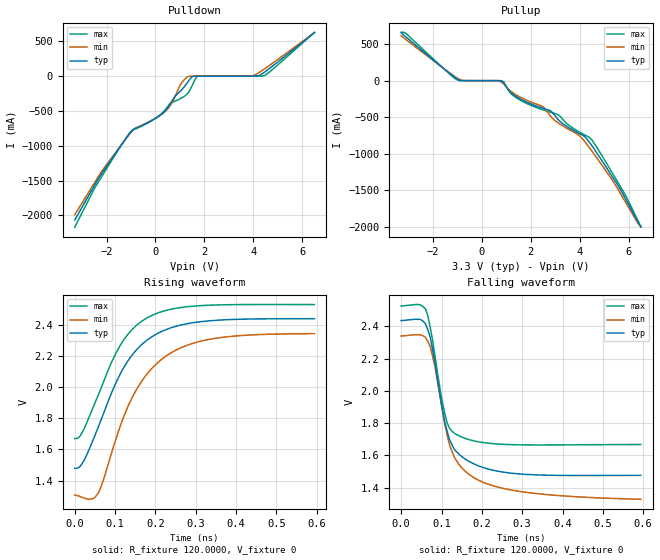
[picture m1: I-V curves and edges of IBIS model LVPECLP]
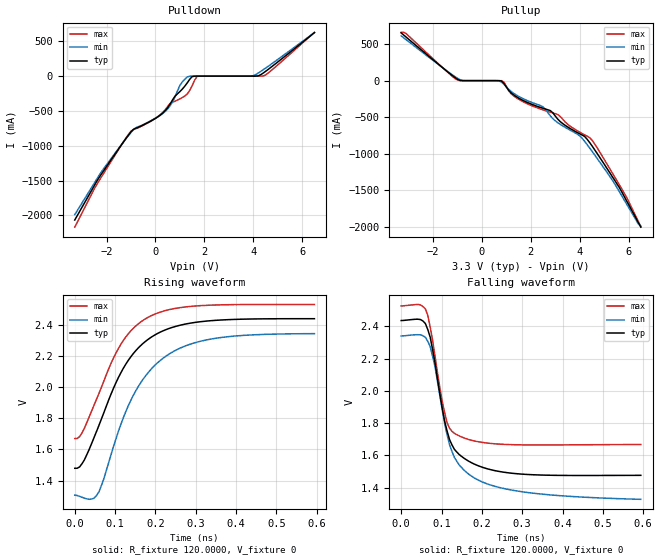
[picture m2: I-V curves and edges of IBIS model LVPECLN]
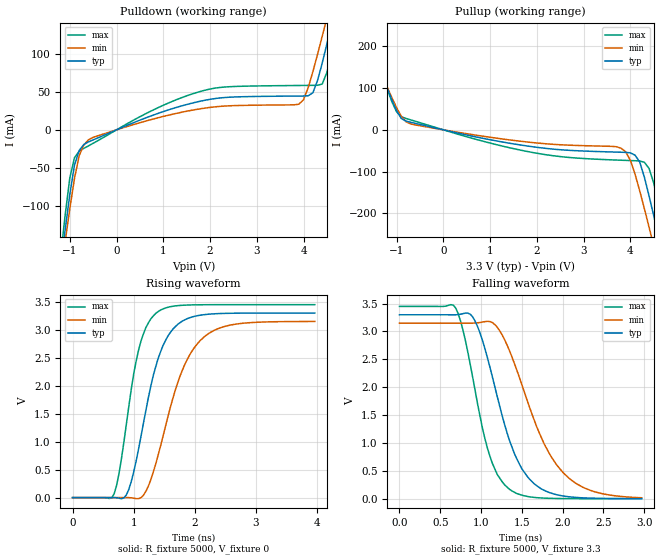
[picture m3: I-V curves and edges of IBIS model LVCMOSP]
|   National Semiconductor Corporation
|   IBIS Model of LMK04000
[IBIS Ver]   4.0
[File name]   lmk04000.ibs
[File Rev]   1.1
[Notes]
 Created By  Shrikant G Kadadevar, Pegah Alavi
   Revision History
   1.0   | Initial Release (SK)
   1.1   | Updated package model per designer's request (PA)
   | Updated pin names & numbers per designer's request (PA)
   | Changed IBIS version from 3.2 to 4.0  (PA)
[Date]   07/09/2009
[Source]  Generated by National Semincoductor Corporation.
[Disclaimer]
(C) Copyright National Semiconductor Corporation 2009
   All rights reserved
National Semiconductor Corporation hereby grants the
user of this IBIS model a non-exclusive, nontransferable
license to use this IBIS model under the following terms.
Before using this IBIS model, the user should read this
license.  If the user does not accept these terms,  the
IBIS model should be returned to National within 30 days.
The user is granted this license only to use the
IBIS model and is not granted rights to sell, load, rent,
lease or license the IBIS model in whole or in part, or in
modified form to anyone other than user. User may modify
the IBIS model to suit its specific applications but rights
to derivative works and such modifications shall belong to
National.
This IBIS model is provided on an "AS IS" basis and
National makes absolutely no warranty with respect to the
information contained herein.NATIONAL DISCLAIMS AND CUSTOMER
WAIVES ALL WARRANTIES, EXPRESS OR IMPLIED, INCLUDING
WARRANTIES OF MERCHANTABILITY OR FITNESS FOR A PARTICULAR
PURPOSE. The entire risk as to quality and performance is
with the Customer. ACCORDINGLY, IN NO EVENT SHALL THE
COMPANY BE LIABLE FOR ANY DAMAGES, WHETHER IN CONTRACT OR
TORT,INCLUDING ANY LOST PROFITS OR OTHER INCIDENTAL,
CONSEQUENTIAL, EXEMPLARY, OR PUNITIVE DAMAGES ARISING OUT
OF THE USE OR APPLICATION OF THE IBIS model provided in
this package.Further, National reserves the right to make
changes without notice to any product herein to improve
reliability, function, or design. National does not convey
any license under patent rights or any other intellectual
property rights, including those of third parties.
National is not obligated to provide maintenance or support
for the licensed IBIS model.
[Copyright]  Copyright 2009, National Semiconductor, All Rights Reserved
[Component]  LMK04000
[Manufacturer]  National Semiconductor Corp
[Package]
|   typ   min   max
R_pkg   0   0   0
L_pkg   0   0   0
C_pkg   0   0   0
[Pin]   signal_name   model_name   R_pin   L_pin   C_pin
1   GND   GND
2   FOUT   NC
3   VCC1   POWER
4   CLKUWIRE   NC
5   DATAUWIRE   NC
6   LEUWIRE   NC
7   NC   NC
8   VCC2   POWER
9   LDOBYP1   POWER
10   LDOBYP2   POWER
11   GOE   NC
12   LD   NC
13   VCC3   POWER
14   CLKOUT0   LVPECLP
15   CLKOUT0*   LVPECLN
16   DLD_BYP   NC
17   GND   POWER
18   VCC4   POWER
19   VCC5   POWER
20   CLKIN0   CLKINP
21   CLKIN0*   CLKINN
22   VCC6   POWER
23   CPOUT1   NC
24   VCC7   POWER
25   CLKIN1   CLKINP
26   CLKIN1*   CLKINN
27   SYNC*   NC
28   OSCIN   OSCINP
29   OSCIN*   OSCINN
30   VCC8   POWER
31   VCC9   POWER
32   CPOUT2   NC
33   VCC10   POWER
34   CLKIN0_LOS   NC
35   CLKIN1_LOS   NC
36   BIAS   NC
37   VCC11   POWER
38   CLKOUT1   LVPECLP
39   CLKOUT1*   LVPECLN
40   VCC12   POWER
41   CLKOUT2   LVCMOSP
42   CLKOUT2*   LVCMOSN
43   VCC13   POWER
44   CLKOUT3   LVCMOSP
45   CLKOUT3*   LVCMOSN
46   VCC14   POWER
47   CLKOUT4   LVPECLP
48   CLKOUT4*   LVPECLN
49   DAP   GND
[Diff pin]  inv_pin  vdiff  tdelay_typ  tdelay_min  tdelay_max
14   15   0.0   0.0s   0.0s   0.0s
20   21   300m   0.0s   0.0s   0.0s
25   26   300m   0.0s   0.0s   0.0s
28   29   300m   0.0s   0.0s   0.0s
38   39   0.0   0.0s   0.0s   0.0s
41   42   0.0   0.0s   0.0s   0.0s
44   45   0.0   0.0s   0.0s   0.0s
47   48   0.0   0.0s   0.0s   0.0s
[Package Model] llp48_lmk04000bisq
[Define Package Model]  llp48_lmk04000bisq
[Manufacturer]  Unknown
[OEM]  Unknown
[Description]  48 LLP for LMK04000 (5GHz simulation Frequency)
[Number Of Pins]  49
[Pin Numbers]
1   | 1 = L1
2   | 2 = L2
3   | 3 = L3
4   | 4 = L4
5   | 5 = L5
6   | 6 = L6
7   | 7 = L7
8   | 8 = L8
9   | 9 = L9
10   | 10 = L10
11   | 11 = L11
12   | 12 = L12
13   | 13 = L13
14   | 14 = L14
15   | 15 = L15
16   | 16 = L16
17   | 17 = L17
18   | 18 = L18
19   | 19 = L19
20   | 20 = L20
21   | 21 = L21
22   | 22 = L22
23   | 23 = L23
24   | 24 = L24
25   | 25 = L25
26   | 26 = L26
27   | 27 = L27
28   | 28 = L28
29   | 29 = L29
30   | 30 = L30
31   | 31 = L31
32   | 32 = L32
33   | 33 = L33
34   | 34 = L34
35   | 35 = L35
36   | 36 = L36
37   | 37 = L37
38   | 38 = L38
39   | 39 = L39
40   | 40 = L40
41   | 41 = L41
42   | 42 = L42
43   | 43 = L43
44   | 44 = L44
45   | 45 = L45
46   | 46 = L46
47   | 47 = L47
48   | 48 = L48
49   | 49 = LDAP
[Model Data]
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[End Model Data]
[End Package Model]
| Models and submodels in the file (8): LVPECLP (Output), LVPECLN (Output), LVCMOSP (Output), LVCMOSN (Output), OSCINP (Input), OSCINN (Input), CLKINP (Input), CLKINN (Input)
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|   Model LVPECLP
[Model]  LVPECLP
Model_type Output
Polarity   Non-Inverting
Vmeas =  1.9572
Rref =   120.0000
Vref =   0
C_comp   1.5000pF   NA   NA
[Temperature Range]   25.0000   85.0000   -40.0000
[Voltage Range]   3.3000V   3.1500V   3.4500V
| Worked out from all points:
|   slope of the pulldown table from 0 to 0.495 V, typ, clamps not added: 3.28 ohm
|   rising waveform, R_fixture 120.0000, V_fixture 0: 20-80 % time 109ps typ, 113ps min, 97ps max; typ from 1.48 V to 2.44 V
|   falling waveform, R_fixture 120.0000, V_fixture 0: 20-80 % time 46.6ps typ, 63.2ps min, 35.4ps max; typ from 2.44 V to 1.48 V
[Pulldown]
|Voltage   I(typ)   I(min)   I(max)
-3.3V     -2.068A    -1.991A    -2.17A
-2.4V     -1.51A     -1.48A     -1.557A
-1V       -800.1mA   -808.9mA   -790.6mA
400mV     -496mA     -506.6mA   -482.6mA
700mV     -340.5mA   -370.2mA   -374.4mA
1V        -221.6mA   -133.2mA   -327mA
1.3V      -96.95mA   -12.44mA   -256.5mA
1.5V      -7.042mA   -45.2uA    -138.2mA
1.7V      -4.607uA   -80.81nA   -4.382mA
4V        8.686uA    6.676mA    32.57pA
4.5V      67.89mA    114.4mA    16.63mA
6.5V      624.9mA    626mA      629.5mA
[Pullup]
|Voltage   I(typ)   I(min)   I(max)
-3.3V     653.2mA    613mA      661mA
-3.1V     596.5mA    561.2mA    645.3mA
-1V       19.76mA    33.01mA    9.085mA
800mV     -4.036mA   -19.24mA   -656.9uA
1.4V      -217.4mA   -195mA     -232mA
2.5V      -377.9mA   -358.4mA   -399.6mA
2.8V      -410.4mA   -481.5mA   -431.5mA
3.1V      -524.8mA   -573.4mA   -462.8mA
4V        -726.7mA   -754.8mA   -705mA
4.4V      -843.3mA   -917.3mA   -777.8mA
5.8V      -1.571A    -1.62A     -1.526A
6.5V      -2.004A    -1.989A    -1.996A
[Ramp]
| variable   typ   min   max
dV/dt_r   563.56m/105.40p   607.29m/112.59p   516.19m/96.90p
dV/dt_f   563.56m/44.92p   607.29m/62.94p   516.19m/35.24p
R_load = 120.00
[Rising Waveform]
R_fixture= 120.0000
V_fixture= 0
|V_fixture_min= 1.8234
|V_fixture_max= 2.0978
|time   V(typ)   V(min)   V(max)
0s        1.479V     1.306V     1.669V
24ps      1.533V     1.287V     1.736V
48ps      1.677V     1.287V     1.885V
60ps      1.754V     1.327V     1.958V
96ps      1.992V     1.618V     2.185V
132ps     2.168V     1.876V     2.338V
192ps     2.323V     2.121V     2.459V
252ps     2.389V     2.237V     2.505V
324ps     2.421V     2.3V       2.523V
594ps     2.437V     2.341V     2.528V
|600.0E-12   2.4373   2.3416   2.5279
[Falling Waveform]
R_fixture= 120.0000
V_fixture= 0
|V_fixture_min= 1.8234
|V_fixture_max= 2.0978
|time   V(typ)   V(min)   V(max)
0s        2.436V     2.34V      2.526V
48ps      2.442V     2.347V     2.533V
66ps      2.38V      2.307V     2.468V
84ps      2.172V     2.147V     2.213V
102ps     1.89V      1.879V     1.931V
114ps     1.749V     1.726V     1.802V
132ps     1.637V     1.587V     1.737V
162ps     1.572V     1.495V     1.703V
288ps     1.486V     1.379V     1.666V
594ps     1.476V     1.328V     1.667V
|   Model LVPECLN
[Model]  LVPECLN
Model_type Output
Polarity   Inverting
Vmeas =  1.9572V
Rref =   120.0000
Vref =   0
C_comp   1.5000pF   NA   NA
[Temperature Range]   25.0000   85.0000   -40.0000
[Voltage Range]   3.3000V   3.1500V   3.4500V
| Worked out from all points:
|   slope of the pulldown table from 0 to 0.495 V, typ, clamps not added: 3.28 ohm
|   rising waveform, R_fixture 120.0000, V_fixture 0: 20-80 % time 109ps typ, 113ps min, 97ps max; typ from 1.48 V to 2.44 V
|   falling waveform, R_fixture 120.0000, V_fixture 0: 20-80 % time 46.6ps typ, 63.2ps min, 35.4ps max; typ from 2.44 V to 1.48 V
[Pulldown]
|Voltage   I(typ)   I(min)   I(max)
-3.3V     -2.068A    -1.991A    -2.17A
-2.4V     -1.51A     -1.48A     -1.557A
-1V       -800.1mA   -808.9mA   -790.6mA
400mV     -496mA     -506.6mA   -482.6mA
700mV     -340.5mA   -370.2mA   -374.4mA
1V        -221.6mA   -133.2mA   -327mA
1.3V      -96.95mA   -12.44mA   -256.5mA
1.5V      -7.042mA   -45.2uA    -138.2mA
1.7V      -4.607uA   -80.81nA   -4.382mA
4V        8.686uA    6.676mA    32.57pA
4.5V      67.89mA    114.4mA    16.63mA
6.5V      624.9mA    626mA      629.5mA
[Pullup]
|Voltage   I(typ)   I(min)   I(max)
-3.3V     653.2mA    613mA      661mA
-3.1V     596.5mA    561.2mA    645.3mA
-1V       19.76mA    33.01mA    9.085mA
800mV     -4.036mA   -19.24mA   -656.9uA
1.4V      -217.4mA   -195mA     -232mA
2.5V      -377.9mA   -358.4mA   -399.6mA
2.8V      -410.4mA   -481.5mA   -431.5mA
3.1V      -524.8mA   -573.4mA   -462.8mA
4V        -726.7mA   -754.8mA   -705mA
4.4V      -843.3mA   -917.3mA   -777.8mA
5.8V      -1.571A    -1.62A     -1.526A
6.5V      -2.004A    -1.989A    -1.996A
[Ramp]
| variable   typ   min   max
dV/dt_r   563.56m/105.40p   607.29m/112.59p   516.19m/96.90p
dV/dt_f   563.56m/44.92p   607.29m/62.94p   516.19m/35.24p
R_load = 120.00
[Rising Waveform]
R_fixture= 120.0000
V_fixture= 0
|V_fixture_min= 1.8234
|V_fixture_max= 2.0978
|time   V(typ)   V(min)   V(max)
0s        1.479V     1.306V     1.669V
24ps      1.533V     1.287V     1.736V
48ps      1.677V     1.287V     1.885V
60ps      1.754V     1.327V     1.958V
96ps      1.992V     1.618V     2.185V
132ps     2.168V     1.876V     2.338V
192ps     2.323V     2.121V     2.459V
252ps     2.389V     2.237V     2.505V
324ps     2.421V     2.3V       2.523V
594ps     2.437V     2.341V     2.528V
|600.0E-12   2.4373   2.3416   2.5279
[Falling Waveform]
R_fixture= 120.0000
V_fixture= 0
|V_fixture_min= 1.8234
|V_fixture_max= 2.0978
|time   V(typ)   V(min)   V(max)
0s        2.436V     2.34V      2.526V
48ps      2.442V     2.347V     2.533V
66ps      2.38V      2.307V     2.468V
84ps      2.172V     2.147V     2.213V
102ps     1.89V      1.879V     1.931V
114ps     1.749V     1.726V     1.802V
132ps     1.637V     1.587V     1.737V
162ps     1.572V     1.495V     1.703V
288ps     1.486V     1.379V     1.666V
594ps     1.476V     1.328V     1.667V
|   Model LVCMOSP
[Model]  LVCMOSP
Model_type Output
Polarity   Non-Inverting
Vmeas =  1.65V
Rref =   50.0000
Vref =   1.65V
C_comp   1.3000pF   NA   NA
[Temperature Range]   25.0000   85.0000   -40.0000
[Voltage Range]   3.3000V   3.1500V   3.4500V
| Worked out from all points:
|   slope of the pulldown table from 0 to 0.495 V, typ, clamps not added: 39.1 ohm
|   slope of the pullup table from 0 to 0.495 V, typ, clamps not added: 40.4 ohm
|   rising waveform, R_fixture 5000, V_fixture 0: 20-80 % time 410ps typ, 533ps min, 311ps max; typ from 0 V to 3.3 V
|   falling waveform, R_fixture 5000, V_fixture 3.3: 20-80 % time 400ps typ, 526ps min, 306ps max; typ from 3.3 V to 0 V
[Pulldown]
|Voltage   I(typ)   I(min)   I(max)
-3.3V     -1.357A    -1.246A    -1.518A
-1.2V     -181.8mA   -193.5mA   -168.5mA
-1.1V     -132mA     -147.7mA   -112.6mA
-900mV    -46.51mA   -64.09mA   -36.69mA
-600mV    -15.8mA    -13.08mA   -21.07mA
1.8V      37.8mA     27.77mA    50.67mA
3.9V      44.52mA    33.75mA    58.41mA
4.2V      48.77mA    76.48mA    58.59mA
4.5V      113.1mA    147.5mA    75.47mA
4.6V      139.3mA    172.4mA    101.3mA
4.8V      193.6mA    225.6mA    159.7mA
6.5V      748.4mA    724.5mA    787mA
[Pullup]
|Voltage   I(typ)   I(min)   I(max)
-3.3V     783.8mA    709.6mA    825.3mA
-1.7V     250.6mA    238.9mA    267mA
-1V       45.55mA    52.6mA     42.93mA
-700mV    18.09mA    14.13mA    23.87mA
1.8V      -38.81mA   -29.18mA   -51.94mA
3.8V      -53.62mA   -43.82mA   -72.76mA
4V        -55.05mA   -72.98mA   -73.57mA
4.2V      -77.23mA   -146.2mA   -74.51mA
4.5V      -206.1mA   -278.3mA   -127.8mA
4.6V      -255.3mA   -324mA     -177.6mA
4.8V      -356.1mA   -417.1mA   -287.9mA
6.5V      -1.305A    -1.248A    -1.356A
[Ramp]
| variable   typ   min   max
dV/dt_r  1.9858/411.52p   1.8870/534.30p   2.0688/310.71p
dV/dt_f  1.9858/401.11p   1.8870/533.17p   2.0688/304.10p
R_load = 50.00
[Rising Waveform]
R_fixture= 5000
V_fixture= 0
V_fixture_min= 0
V_fixture_max= 0
|time   V(typ)   V(min)   V(max)
0s        1.87uV     2.13uV     1.614uV
680ps     194.6uV    -21.12uV   66.83mV
760ps     -11.43mV   55.75uV    434.4mV
920ps     147.1mV    -871.5uV   1.632V
1.12ns    1.101V     -1.119mV   2.804V
1.36ns    2.341V     602.6mV    3.294V
1.56ns    2.891V     1.45V      3.403V
1.76ns    3.13V      2.182V     3.437V
2.16ns    3.272V     2.881V     3.449V
3.96ns    3.3V       3.149V     3.45V
|4.0E-9   3.3000   3.1495   3.4500
[Falling Waveform]
R_fixture= 5000
V_fixture= 3.3
V_fixture_min= 3.15
V_fixture_max= 3.45
|time   V(typ)   V(min)   V(max)
0s        3.3V       3.15V      3.45V
690ps     3.3V       3.15V      3.42V
810ps     3.33V      3.15V      2.83V
960ps     3.082V     3.156V     1.688V
1.14ns    2.184V     3.159V     633mV
1.35ns    1.043V     2.652V     167.8mV
1.59ns    358.5mV    1.663V     34.51mV
2.01ns    48.26mV    462.2mV    2.128mV
2.4ns     7.178mV    122mV      164.5uV
2.97ns    447.9uV    16.38mV    5.603uV
